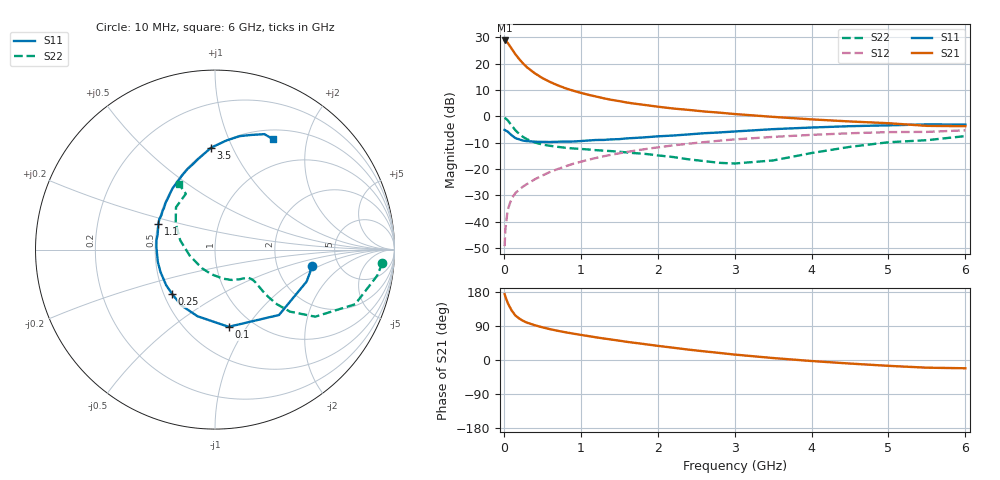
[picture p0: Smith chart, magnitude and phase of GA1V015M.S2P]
! Infineon Technologies  Discrete & RF Semiconductors
! BF775
! Si NPN RF Bipolar Junction Transistor in SOT23
! VCE = 1 V  IC = 15 mA
! Common Emitter S-Parameters:  May  1996
# GHz  S  MA  R  50
!  f  S11  S21  S12  S22
! GHz  MAG  ANG  MAG  ANG  MAG  ANG  MAG  ANG
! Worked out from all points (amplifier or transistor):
!   36 points, 10 MHz to 6 GHz, reference 50 ohm
!   highest |S21| = 28.8 dB at 10 MHz (marker M1)
!   |S21| within 3 dB of that: start of sweep to 98.72 MHz
!   unconditionally stable (mu >= 1): 325.7 MHz to end of sweep
!   at 250 MHz: K = 0.90, MSG = 23.4 dB, |S12| = -26.7 dB
!   at 1.4 GHz: K = 1.21, MAG = 7.7 dB, |S12| = -14.6 dB
!   at 6 GHz: K = 1.05, MAG = -0.6 dB, |S12| = -5.4 dB
!   S11 on the Smith chart (normalised r, x): 10 MHz: 3.19, -0.86; 100 MHz: 0.78, -0.83; 250 MHz: 0.55, -0.31; 1.1 GHz: 0.50, +0.16; 3.5 GHz: 0.50, +0.83; 6 GHz: 0.62, +1.48
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0.01  0.5498 -9.8  27.51 173.8  0.0034 85.0  0.9358 -4.5
0.02  0.5407 -19.2  27.08 167.4  0.0071 83.4  0.9154 -9.1
0.05  0.5099 -45.6  24.78 151.0  0.0166 72.7  0.8382 -21.3
0.1  0.4368 -80.0  19.35 131.1  0.0271 63.2  0.6718 -33.8
0.15  0.384 -104.7  15.05 117.6  0.0347 60.0  0.5422 -39.6
0.2  0.3631 -121.3  12.16 109.5  0.0403 59.6  0.4603 -41.4
0.25  0.3435 -134.1  10.04 103.3  0.0461 60.4  0.404 -41.6
0.3  0.3368 -143.9  8.525 98.6  0.0515 61.9  0.3659 -41.3
0.4  0.3283 -158.1  6.581 91.9  0.0631 63.3  0.3182 -40.0
0.5  0.3258 -167.9  5.314 86.3  0.0747 64.6  0.2903 -39.0
0.6  0.324 -176.5  4.478 81.4  0.0872 64.9  0.2743 -38.7
0.7  0.3276 176.6  3.871 77.1  0.099 65.2  0.2622 -39.0
0.8  0.3302 171.0  3.404 73.2  0.1116 64.6  0.2519 -39.5
1.1  0.3457 155.8  2.553 63.1  0.149 62.7  0.2332 -43.4
1.3  0.3547 147.5  2.191 56.7  0.1738 60.7  0.2217 -46.9
1.6  0.3795 136.5  1.82 47.9  0.2098 57.2  0.2048 -54.4
2.2  0.43 119.4  1.402 32.4  0.2791 49.3  0.1679 -74.8
3  0.5131 100.6  1.101 14.3  0.3625 37.7  0.1265 -125.0
3.5  0.5682 92.2  0.972 5.2  0.4053 30.3  0.1445 -166.3
4.5  0.6471 77.7  0.795 -9.4  0.475 16.2  0.2621 146.6
5.5  0.6998 66.8  0.656 -20.3  0.504 2.3  0.3506 117.6
6  0.6947 62.1  0.647 -21.8  0.54 -1.7  0.4195 118.9
